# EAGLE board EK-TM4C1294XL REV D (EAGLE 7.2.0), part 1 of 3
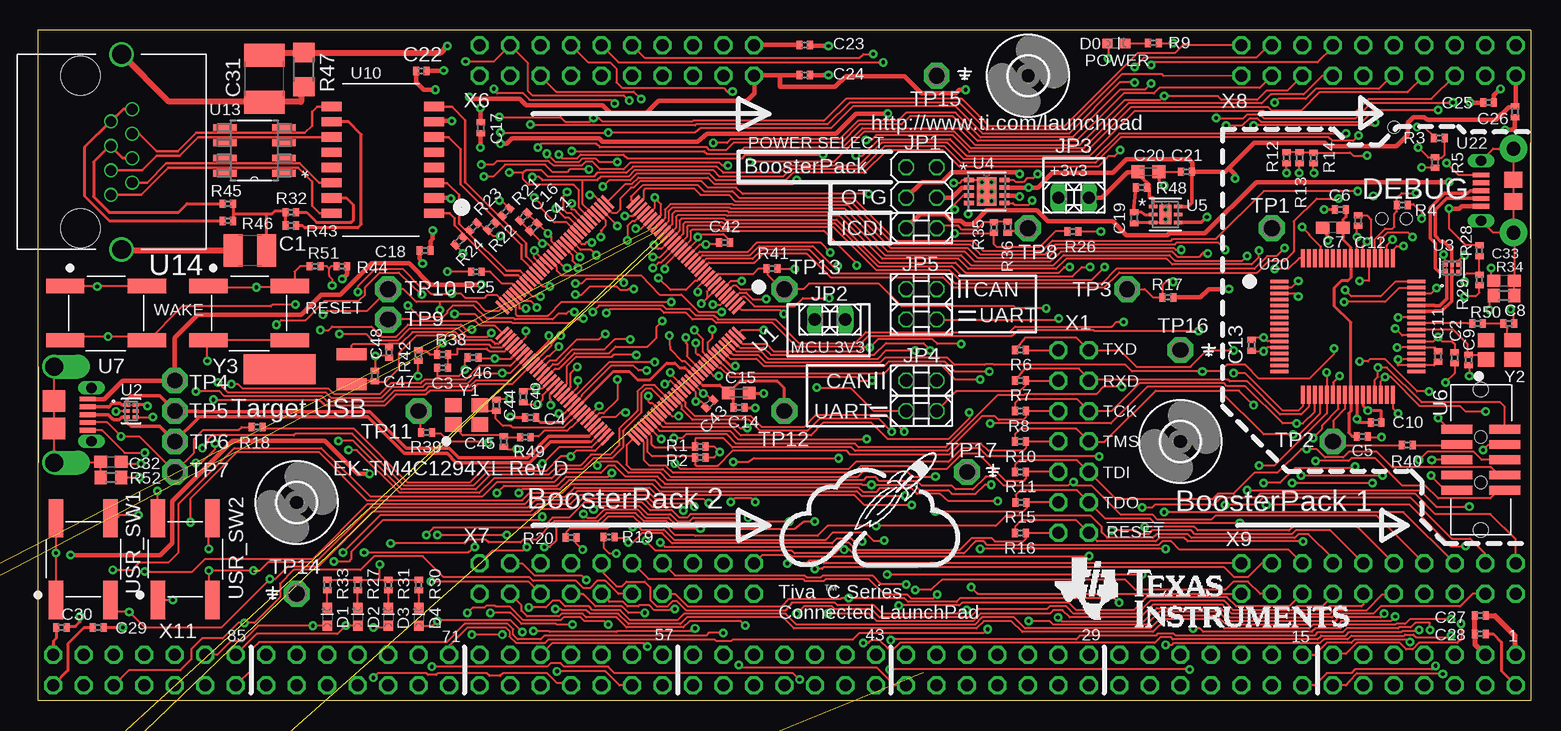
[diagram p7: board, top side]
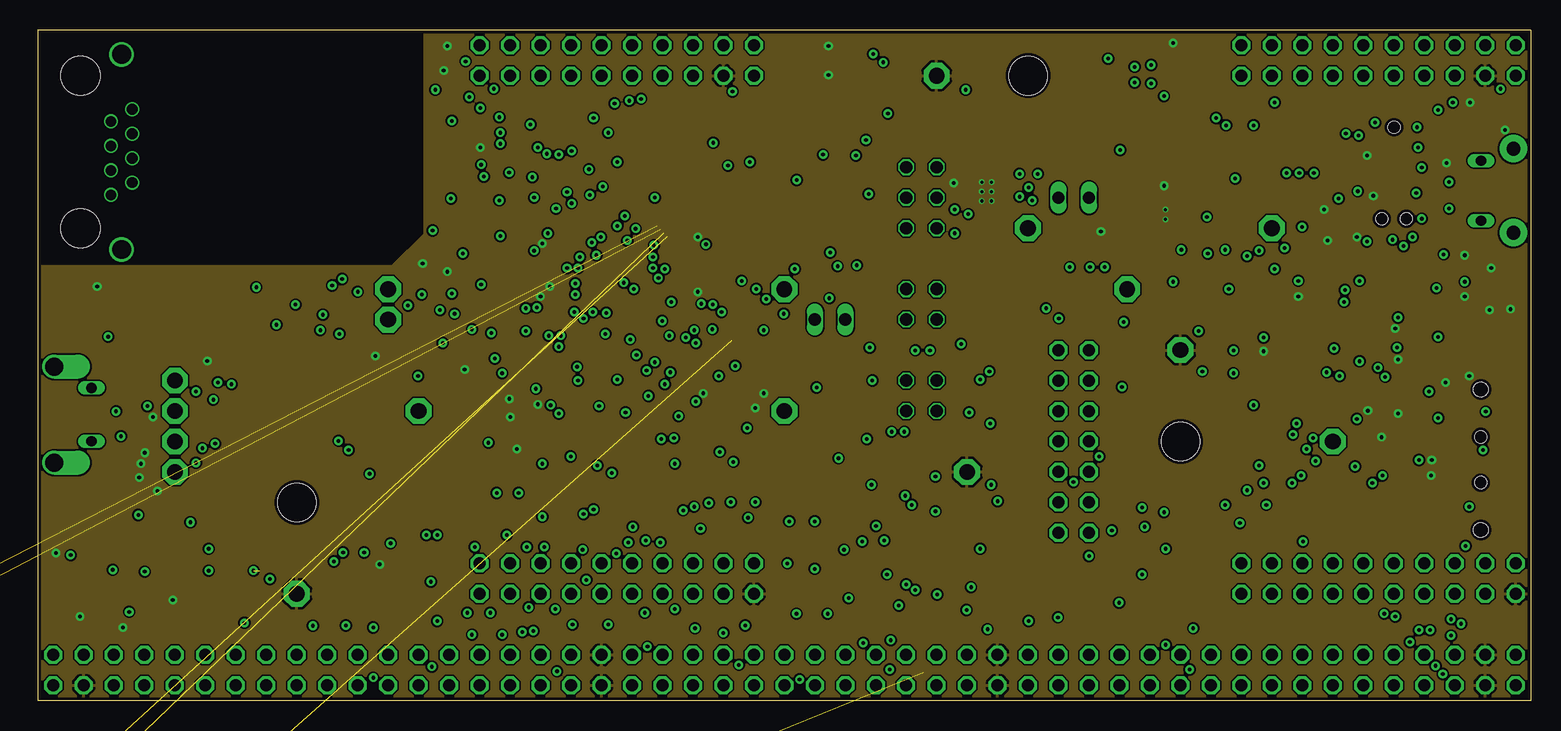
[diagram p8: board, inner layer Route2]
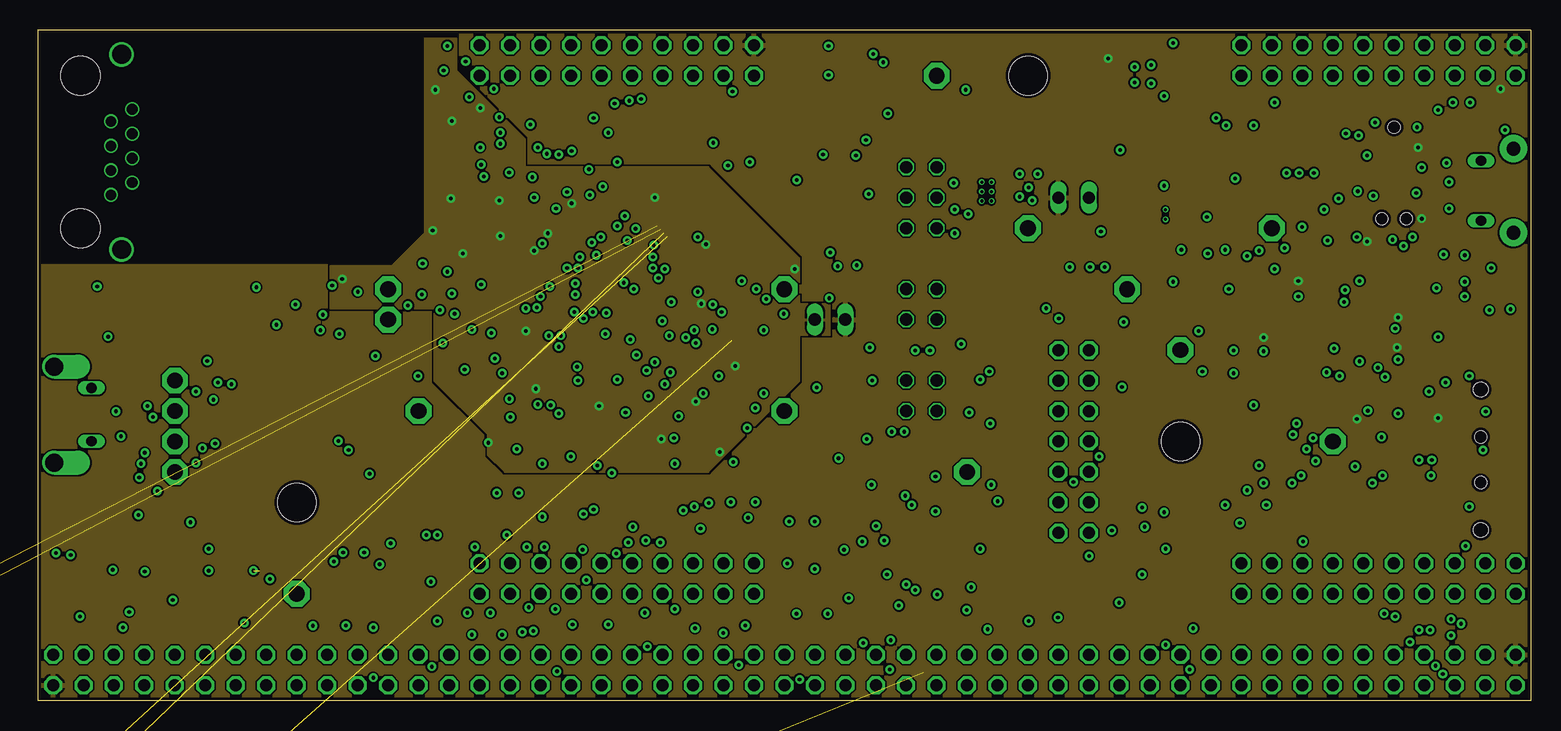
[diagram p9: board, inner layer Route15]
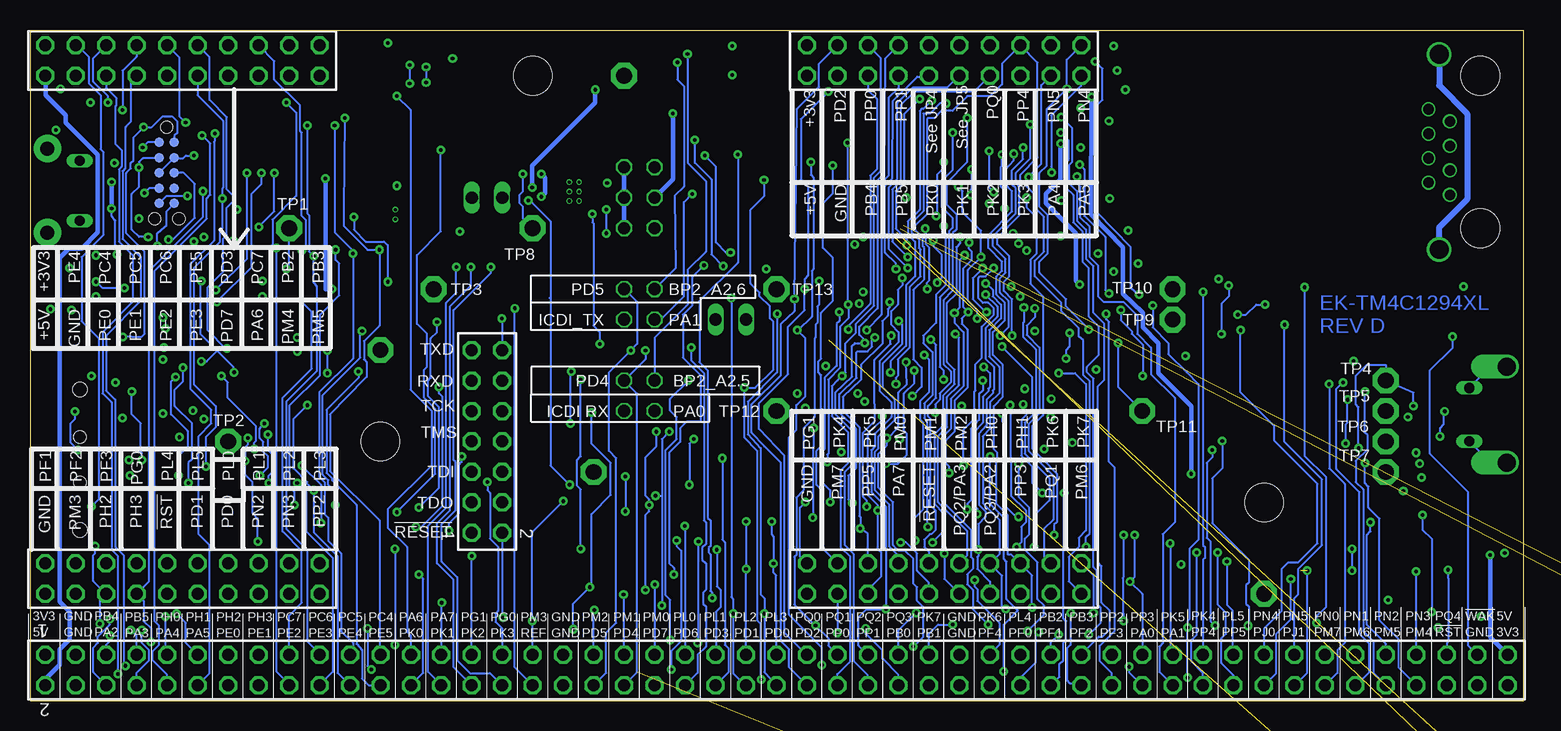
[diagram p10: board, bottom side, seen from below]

Size 124.46 x 55.88 mm. Coordinates in mm from the lower left corner, seen from the top.
Outline: 124.46,55.88 124.46,0 0,0 0,55.88 124.46,55.88
Copper layers (1+2*15+16): Top 0.035mm / dielectric 0.22mm / Route2 0.035mm / dielectric 1mm / Route15 0.035mm / dielectric 0.22mm / Bottom 0.035mm
Design rules "default *": minimum track width 6mil, minimum drill 12mil, track to track 6mil, track to pad 6mil, pad to pad 5mil, via to via 6mil, smd to smd 5mil, copper to edge 10mil, drill to drill 8mil, minimum pad ring 4mil, minimum via ring 8mil, stop-mask expansion 2mil, vias tented up to drill 13mil, thermal gap 8mil
Net classes: 1 USB: width 0.275 mm, clearance 0.152 mm; 2 Ethernet: width 0.22 mm, clearance 0.152 mm

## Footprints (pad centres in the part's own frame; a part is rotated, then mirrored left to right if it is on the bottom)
C1210 = smd 1.6 x 2.7: 1 -1.4,0; 2 1.4,0
C0402 = smd 0.5 x 0.7: 1 -0.45,0; 2 0.45,0
C0603 = smd 1.1 x 1: 1 -0.85,0; 2 0.85,0
C0603K = smd 1.05 x 1.08: 1 -0.875,0; 2 0.875,0
C1812 = smd 1.9 x 3.4: 1 -1.95,0; 2 1.95,0
CHIPLED_0603 = smd 0.8 x 0.8: A 0,-0.75; C 0,0.75
3,2 = hole 3.2: 0,0
2X03 = drill 1.016 octagon: 1 -2.54,-1.27; 2 -2.54,1.27; 3 0,-1.27; 4 0,1.27; 5 2.54,-1.27; 6 2.54,1.27
1X02 = drill 1.016 long: 1 -1.27,0; 2 1.27,0
2X02 = drill 1.016 octagon: 1 -1.27,-1.27; 2 -1.27,1.27; 3 1.27,-1.27; 4 1.27,1.27
R0402 = smd 0.5 x 0.7: 1 -0.45,0; 2 0.45,0
R0603 = smd 1 x 1.1: 1 -0.85,0; 2 0.85,0
R1206 = smd 1.6 x 1.803: 1 -1.422,0; 2 1.422,0
SWITCH_6MM_6MM_TE_CON_SMD = smd 1.2 x 3.2: P$1 4.521,6.807; P$2 4.521,0; P$3 0,6.807; P$4 0,0
P1-13 = drill 1.321 pad 2.159 octagon: TP 0,0
TQFP-128 = smd 1.45 x 0.25: P$1 0,0; P$2 0,-0.4; P$3 0,-0.8; P$4 0,-1.2; P$5 0,-1.6; P$6 0,-2; P$7 0,-2.4; P$8 0,-2.8; P$9 0,-3.2; P$10 0,-3.6; P$11 0,-4; P$12 0,-4.4; P$13 0,-4.8; P$14 0,-5.2; P$15 0,-5.6; P$16 0,-6; P$17 0,-6.4; P$18 0,-6.8; P$19 0,-7.2; P$20 0,-7.6; P$21 0,-8; P$22 0,-8.4; P$23 0,-8.8; P$24 0,-9.2; P$25 0,-9.6; P$26 0,-10; P$27 0,-10.4; P$28 0,-10.8; P$29 0,-11.2; P$30 0,-11.6; P$31 0,-12; P$32 0,-12.4; P$65 15.45,-12.4; P$66 15.45,-12; P$67 15.45,-11.6; P$68 15.45,-11.2; P$69 15.45,-10.8; P$70 15.45,-10.4; P$71 15.45,-10; P$72 15.45,-9.6; P$73 15.45,-9.2; P$74 15.45,-8.8; P$75 15.45,-8.4; P$76 15.45,-8; P$77 15.45,-7.6; P$78 15.45,-7.2; P$79 15.45,-6.8; P$80 15.45,-6.4; P$81 15.45,-6; P$82 15.45,-5.6; P$83 15.45,-5.2; P$84 15.45,-4.8; P$85 15.45,-4.4; P$86 15.45,-4; P$87 15.45,-3.6; P$88 15.45,-3.2; P$89 15.45,-2.8; P$90 15.45,-2.4; P$91 15.45,-2; P$92 15.45,-1.6; P$93 15.45,-1.2; P$94 15.45,-0.8; P$95 15.45,-0.4; P$96 15.45,0 | smd 0.25 x 1.45: P$33 1.525,-13.925; P$34 1.925,-13.925; P$35 2.325,-13.925; P$36 2.725,-13.925; P$37 3.125,-13.925; P$38 3.525,-13.925; P$39 3.925,-13.925; P$40 4.325,-13.925; P$41 4.725,-13.925; P$42 5.125,-13.925; P$43 5.525,-13.925; P$44 5.925,-13.925; P$45 6.325,-13.925; P$46 6.725,-13.925; P$47 7.125,-13.925; P$48 7.525,-13.925; P$49 7.925,-13.925; P$50 8.325,-13.925; P$51 8.725,-13.925; P$52 9.125,-13.925; P$53 9.525,-13.925; P$54 9.925,-13.925; P$55 10.325,-13.925; P$56 10.725,-13.925; P$57 11.125,-13.925; P$58 11.525,-13.925; P$59 11.925,-13.925; P$60 12.325,-13.925; P$61 12.725,-13.925; P$62 13.125,-13.925; P$63 13.525,-13.925; P$64 13.925,-13.925; P$97 13.925,1.525; P$98 13.525,1.525; P$99 13.125,1.525; P$100 12.725,1.525; P$101 12.325,1.525; P$102 11.925,1.525; P$103 11.525,1.525; P$104 11.125,1.525; P$105 10.725,1.525; P$106 10.325,1.525; P$107 9.925,1.525; P$108 9.525,1.525; P$109 9.125,1.525; P$110 8.725,1.525; P$111 8.325,1.525; P$112 7.925,1.525; P$113 7.525,1.525; P$114 7.125,1.525; P$115 6.725,1.525; P$116 6.325,1.525; P$117 5.925,1.525; P$118 5.525,1.525; P$119 5.125,1.525; P$120 4.725,1.525; P$121 4.325,1.525; P$122 3.925,1.525; P$123 3.525,1.525; P$124 3.125,1.525; P$125 2.725,1.525; P$126 2.325,1.525; P$127 1.925,1.525; P$128 1.525,1.525
DRY6 = smd 0.559 x 0.305: 1 -0.356,0.508 | smd 0.508 x 0.305: 2 -0.381,0; 3 -0.381,-0.508; 4 0.381,-0.508; 5 0.381,0; 6 0.381,0.508
DRB8_2P4X1P65 = smd 0.838 x 0.356: 1 -1.473,0.965; 2 -1.473,0.33; 3 -1.473,-0.33; 4 -1.473,-0.965; 5 1.473,-0.965; 6 1.473,-0.33; 7 1.473,0.33; 8 1.473,0.965 | smd 1.651 x 2.388: 9 0,0 | drill 0.254: V 0.406,0.787; V_2 -0.406,0; V_3 -0.406,-0.787; V_4 -0.406,0.787; V_5 0.406,-0.787; V_6 0.406,0
DRV6_1P6X1 = smd 0.711 x 0.305: 1 -1.041,0.66; 2 -1.041,0; 3 -1.041,-0.66; 4 1.041,-0.66; 5 1.041,0; 6 1.041,0.66 | smd 1.016 x 1.6: 7 0,0 | drill 0.254: V 0,-0.406; V_2 0,0.406
CON_2X5_50MIL = smd 0.74 x 2.6: P1 0,0; P2 0,4.008; P3 1.27,0; P4 1.27,4.008; P5 2.54,0; P6 2.54,4.008; P7 3.81,0; P8 3.81,4.008; P9 5.08,0; P10 5.08,4.008 | hole 1: 4.44,2; 0.64,2 | hole 1.2: 8.407,2; -3.327,2
CON_USB_MICRO_AB_HIROSE_ZX62D-AB-5P8 = smd 1.35 x 0.4: P1 2.8,1.3; P2 2.8,0.65; P3 2.8,0; P4 2.8,-0.65; P5 2.8,-1.3 | smd 1.9 x 1.8: P$1 0,-1.15; P$2 0,1.15 | drill 0.85 pad 1.092 long: P$3 3.125,2.225; P$4 3.125,-2.225 | drill 1.5 pad 2 offset: P$5 0,-4; P$6 0,4
DIL28-3 = drill 0.813 long: 1 -16.51,-3.81; 2 -13.97,-3.81; 3 -11.43,-3.81; 4 -8.89,-3.81; 5 -6.35,-3.81; 6 -3.81,-3.81; 7 -1.27,-3.81; 8 1.27,-3.81; 9 3.81,-3.81; 10 6.35,-3.81; 11 8.89,-3.81; 12 11.43,-3.81; 13 13.97,-3.81; 14 16.51,-3.81; 15 16.51,3.81; 16 13.97,3.81; 17 11.43,3.81; 18 8.89,3.81; 19 6.35,3.81; 20 3.81,3.81; 21 1.27,3.81; 22 -1.27,3.81; 23 -3.81,3.81; 24 -6.35,3.81; 25 -8.89,3.81; 26 -11.43,3.81; 27 -13.97,3.81; 28 -16.51,3.81
MAG_PULSE_HX1188FNL = smd 0.76 x 1.67: P$1 0,0; P$2 1.27,0; P$3 2.54,0; P$4 3.81,0; P$5 5.08,0; P$6 6.35,0; P$7 7.62,0; P$8 8.89,0; P$9 8.89,8.55; P$10 7.62,8.55; P$11 6.35,8.55; P$12 5.08,8.55; P$13 3.81,8.55; P$14 2.54,8.55; P$15 1.27,8.55; P$16 0,8.55
BLUETOOTH_SMD = smd 2 x 1: 1 0,0; 2 0,-1.5; 3 0,-3; 4 0,-4.5; 5 0,-6; 6 0,-7.5; 7 0,-9; 8 0,-10.5; 9 0,-12; 10 0,-13.5; 11 0,-15; 12 0,-16.5; 13 0,-18; 22 13,-18; 23 13,-16.5; 24 13,-15; 25 13,-13.5; 26 13,-12; 27 13,-10.5; 28 13,-9; 29 13,-7.5; 30 13,-6; 31 13,-4.5; 32 13,-3; 33 13,-1.5; 34 13,0 | smd 1 x 1.8: 14 1.25,-19.75; 15 2.75,-19.75; 16 4.25,-19.75; 17 5.75,-19.75; 18 7.25,-19.75; 19 8.75,-19.75; 20 10.25,-19.75; 21 11.75,-19.75
D8 = smd 1.981 x 0.559: 1 -2.464,1.905; 2 -2.464,0.635; 3 -2.464,-0.635; 4 -2.464,-1.905; 5 2.464,-1.905; 6 2.464,-0.635; 7 2.464,0.635; 8 2.464,1.905
RJ45_TE_CON_NOMAG_NOLED = drill 0.89: 1 9.93,2.54; 2 8.91,4.32; 3 7.89,2.54; 4 6.87,4.32; 5 5.85,2.54; 6 4.83,4.32; 7 3.81,2.54; 8 2.79,4.32 | drill 1.57: 9 -1.78,3.43; 10 14.48,3.43 | hole 3.25: 0,0; 12.7,0
LQFP-64-PM = smd 1.5 x 0.3: P$1 0,0; P$2 0,-0.5; P$3 0,-1; P$4 0,-1.5; P$5 0,-2; P$6 0,-2.5; P$7 0,-3; P$8 0,-3.5; P$9 0,-4; P$10 0,-4.5; P$11 0,-5; P$12 0,-5.5; P$13 0,-6; P$14 0,-6.5; P$15 0,-7; P$16 0,-7.5; P$33 11.4,-7.5; P$34 11.4,-7; P$35 11.4,-6.5; P$36 11.4,-6; P$37 11.4,-5.5; P$38 11.4,-5; P$39 11.4,-4.5; P$40 11.4,-4; P$41 11.4,-3.5; P$42 11.4,-3; P$43 11.4,-2.5; P$44 11.4,-2; P$45 11.4,-1.5; P$46 11.4,-1; P$47 11.4,-0.5; P$48 11.4,0 | smd 0.3 x 1.5: P$17 1.95,-9.45; P$18 2.45,-9.45; P$19 2.95,-9.45; P$20 3.45,-9.45; P$21 3.95,-9.45; P$22 4.45,-9.45; P$23 4.95,-9.45; P$24 5.45,-9.45; P$25 5.95,-9.45; P$26 6.45,-9.45; P$27 6.95,-9.45; P$28 7.45,-9.45; P$29 7.95,-9.45; P$30 8.45,-9.45; P$31 8.95,-9.45; P$32 9.45,-9.45; P$49 9.45,1.95; P$50 8.95,1.95; P$51 8.45,1.95; P$52 7.95,1.95; P$53 7.45,1.95; P$54 6.95,1.95; P$55 6.45,1.95; P$56 5.95,1.95; P$57 5.45,1.95; P$58 4.95,1.95; P$59 4.45,1.95; P$60 3.95,1.95; P$61 3.45,1.95; P$62 2.95,1.95; P$63 2.45,1.95; P$64 1.95,1.95
TC2030-MCP-NL = smd 0.787 x 0.787: 1 1.27,-0.635; 2 2.54,-0.635; 3 3.81,-0.635; 4 5.08,-0.635; 5 6.35,-0.635; 6 6.35,0.635; 7 5.08,0.635; 8 3.81,0.635; 9 2.54,0.635; 10 1.27,0.635 | hole 1: 0,0; 7.62,-1.016; 7.62,1.016
CON_USB_MICRO_B_FCI_10118194 = smd 1.35 x 0.4: P1 2.7,1.3; P2 2.7,0.65; P3 2.7,0; P4 2.7,-0.65; P5 2.7,-1.3 | smd 1.5 x 1.35: P6 0,0.9; P7 0,-0.9 | drill 0.85 long: P8 2.7,2.5; P9 2.7,-2.5 | drill 1.15 pad 2.286: P10 0,-3.5; P11 0,3.5
TSW-107-02-S-D = drill 1 pad 1.5 octagon: 1 7.62,-1.27; 2 7.62,1.27; 3 5.08,-1.27; 4 5.08,1.27; 5 2.54,-1.27; 6 2.54,1.27; 7 0,-1.27; 8 0,1.27; 9 -2.54,-1.27; 10 -2.54,1.27; 11 -5.08,-1.27; 12 -5.08,1.27; 13 -7.62,-1.27; 14 -7.62,1.27
TSW-110-02-S-D = drill 1 pad 1.5 octagon: 1 11.43,-1.27; 2 11.43,1.27; 3 8.89,-1.27; 4 8.89,1.27; 5 6.35,-1.27; 6 6.35,1.27; 7 3.81,-1.27; 8 3.81,1.27; 9 1.27,-1.27; 10 1.27,1.27; 11 -1.27,-1.27; 12 -1.27,1.27; 13 -3.81,-1.27; 14 -3.81,1.27; 15 -6.35,-1.27; 16 -6.35,1.27; 17 -8.89,-1.27; 18 -8.89,1.27; 19 -11.43,-1.27; 20 -11.43,1.27
TSW-149-02-S-D = drill 1 pad 1.5 octagon: 1 60.96,-1.27; 2 60.96,1.27; 3 58.42,-1.27; 4 58.42,1.27; 5 55.88,-1.27; 6 55.88,1.27; 7 53.34,-1.27; 8 53.34,1.27; 9 50.8,-1.27; 10 50.8,1.27; 11 48.26,-1.27; 12 48.26,1.27; 13 45.72,-1.27; 14 45.72,1.27; 15 43.18,-1.27; 16 43.18,1.27; 17 40.64,-1.27; 18 40.64,1.27; 19 38.1,-1.27; 20 38.1,1.27; 21 35.56,-1.27; 22 35.56,1.27; 23 33.02,-1.27; 24 33.02,1.27; 25 30.48,-1.27; 26 30.48,1.27; 27 27.94,-1.27; 28 27.94,1.27; 29 25.4,-1.27; 30 25.4,1.27; 31 22.86,-1.27; 32 22.86,1.27; 33 20.32,-1.27; 34 20.32,1.27; 35 17.78,-1.27; 36 17.78,1.27; 37 15.24,-1.27; 38 15.24,1.27; 39 12.7,-1.27; 40 12.7,1.27; 41 10.16,-1.27; 42 10.16,1.27; 43 7.62,-1.27; 44 7.62,1.27; 45 5.08,-1.27; 46 5.08,1.27; 47 2.54,-1.27; 48 2.54,1.27; 49 0,-1.27; 50 0,1.27; 51 -2.54,-1.27; 52 -2.54,1.27; 53 -5.08,-1.27; 54 -5.08,1.27; 55 -7.62,-1.27; 56 -7.62,1.27; 57 -10.16,-1.27; 58 -10.16,1.27; 59 -12.7,-1.27; 60 -12.7,1.27; 61 -15.24,-1.27; 62 -15.24,1.27; 63 -17.78,-1.27; 64 -17.78,1.27; 65 -20.32,-1.27; 66 -20.32,1.27; 67 -22.86,-1.27; 68 -22.86,1.27; 69 -25.4,-1.27; 70 -25.4,1.27; 71 -27.94,-1.27; 72 -27.94,1.27; 73 -30.48,-1.27; 74 -30.48,1.27; 75 -33.02,-1.27; 76 -33.02,1.27; 77 -35.56,-1.27; 78 -35.56,1.27; 79 -38.1,-1.27; 80 -38.1,1.27; 81 -40.64,-1.27; 82 -40.64,1.27; 83 -43.18,-1.27; 84 -43.18,1.27; 85 -45.72,-1.27; 86 -45.72,1.27; 87 -48.26,-1.27; 88 -48.26,1.27; 89 -50.8,-1.27; 90 -50.8,1.27; 91 -53.34,-1.27; 92 -53.34,1.27; 93 -55.88,-1.27; 94 -55.88,1.27; 95 -58.42,-1.27; 96 -58.42,1.27; 97 -60.96,-1.27; 98 -60.96,1.27
NDK3.2X2.5 = smd 1.4 x 1.2: P$1 0,0; P$2 2.2,0; P$3 2.2,1.6; P$4 0,1.6
CRYSTAL_32K_SMD = smd 2.5 x 1: P$1 0,1.25; P$2 0,-1.25 | smd 6 x 2.5: P$3 -6,0

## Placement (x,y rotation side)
C1  1000pF  [C1210]  17.68,37.49 180 top
C2  0.1uF  [C0402]  118.11,28.57 270 top
C3  0.1uF  [C0402]  33.76,27.74 180 top
C4  0.1uF  [C0402]  41.07,23.6 180 top
C5  0.1uF  [C0402]  110.41,22 0 top
C6  1.0uF  [C0402]  108.58,40.92 180 top
C7  2.2uF  [C0603]  107.95,39.42 180 top
C8  12pF  [C0402]  122.63,31.42 0 top
C9  12pF  [C0402]  119.25,28.37 270 top
C10  0.1uF  [C0402]  111.56,23.16 0 top
C11  0.1uF  [C0402]  116.71,28.68 270 top
C12  0.1uF  [C0402]  110.06,40.01 270 top
C13  0.1uF  [C0402]  101.17,29.62 270 top
C14  1.0uF  [C0402]  58.45,24.41 0 top
C15  2.2uF  [C0603K]  58.45,25.63 0 top
C16  0.1uF  [C0402]  40.49,40.31 225 top
C17  0.1uF  [C0402]  36.93,47.73 270 top
C18  0.1uF  [C0402]  32.28,37.49 180 top
C19  0.1uF  [C0402]  91.39,40.23 270 top
C20  2.2uF  [C0603K]  92.58,44.07 0 top
C21  0.1uF  [C0402]  95.76,44.07 180 top
C22  0.1uF  [C0402]  31.98,52.48 0 top
C23  0.1uF  [C0402]  63.93,54.64 0 top
C24  0.1uF  [C0402]  63.93,52.12 0 top
C25  0.1uF  [C0402]  120.93,49.83 180 top
C26  0.1uF  [C0402]  123.14,49.07 270 top
C27  0.1uF  [C0402]  120.24,7.09 180 top
C28  0.1uF  [C0402]  120.24,5.56 180 top
C29  0.1uF  [C0402]  5.03,6.1 0 top
C30  0.1uF  [C0402]  1.98,6.1 0 top
C31  4700pF  [C1812]  18.9,51.82 90 top
C32  3300pF  [C0603]  6.1,19.89 0 top
C33  3300pF  [C0603]  122.22,34.98 180 top
C40  0.1uF  [C0402]  40.46,25.32 270 top
C41  0.1uF  [C0402]  41.33,39.45 225 top
C42  0.1uF  [C0402]  57.25,38.18 0 top
C43  0.1uF  [C0402]  56.01,24.74 45 top
C44  12pF  [C0402]  38.23,24.61 90 top
C45  12pF  [C0402]  38.84,21.59 270 top
C46  0.1uF  [C0402]  36.3,28.6 180 top
C47  12pF  [C0402]  28.09,27.05 90 top
C48  12pF  [C0402]  29.29,29.01 270 top
D0  [CHIPLED_0603]  89.92,54.76 270 top
D1  [CHIPLED_0603]  24.13,6.99 0 top
D2  [CHIPLED_0603]  26.67,6.99 0 top
D3  [CHIPLED_0603]  29.21,6.99 0 top
D4  [CHIPLED_0603]  31.75,6.99 0 top
H1  MOUNT-HOLE3.2  [3,2]  95.25,21.59 0 top
H4  MOUNT-HOLE3.2  [3,2]  21.59,16.51 0 top
H6  MOUNT-HOLE3.2  [3,2]  82.55,52.07 0 top
J1  [JUMP]  73.66,39.37 90 top
J2  [JUMP]  73.66,24.13 90 top
J3  [JUMP]  86.36,41.91 90 top
J4  [JUMP]  73.66,26.67 90 top
J5  [JUMP]  73.66,31.75 90 top
J6  [JUMP]  73.66,34.29 90 top
J7  [JUMP]  66.04,31.75 90 top
JP1  [2X03]  73.66,41.91 270 top
JP2  [1X02]  66.04,31.75 180 top
JP3  [1X02]  86.36,41.91 0 top
JP4  [2X02]  73.66,25.4 90 top
JP5  [2X02]  73.66,33.02 90 top
R1  10k  [R0402]  55.22,21.18 180 top
R2  10k  [R0402]  55.22,20.24 180 top
R3  10k  [R0402]  116.84,46.89 0 top
R4  10k  [R0402]  113.74,41.3 180 top
R5  10k  [R0402]  116.48,44.83 270 top
R6  0  [R0402]  81.92,29.21 180 top
R7  0  [R0402]  81.92,26.67 180 top
R8  0  [R0402]  81.92,24.13 180 top
R9  330  [R0402]  92.99,54.81 180 top
R10  0  [R0402]  81.92,21.59 180 top
R11  0  [R0402]  81.92,19.05 180 top
R12  5.6k  [R0402]  104.09,45.24 90 top
R13  5.6k  [R0402]  105.18,45.24 90 top
R14  5.6k  [R0402]  106.35,45.21 90 top
R15  0  [R0402]  81.97,16.51 180 top
R16  0  [R0402]  81.92,13.97 180 top
R17  100k  [R0402]  94.21,33.6 180 top
R18  100  [R0402]  18.29,22.78 180 top
R19  0  [R0402]  47.62,13.61 0 top
R20  0  [R0402]  44.45,13.59 180 top
R21  49.9  [R0402]  39.01,40.72 225 top
R22  49.9  [R0402]  37.82,39.52 45 top
R23  49.4  [R0402]  36.3,39.47 225 top
R24  49.9  [R0402]  35.1,38.28 45 top
R25  4.87k 1%  [R0402]  36.55,35.74 180 top
R26  100k  [R0402]  86.28,39.09 0 top
R27  330  [R0402]  26.67,9.63 270 top
R28  5.6k  [R0402]  120.17,37.49 90 top
R29  10k  [R0402]  120.17,35.05 90 top
R30  330  [R0402]  31.75,9.63 270 top
R31  330  [R0402]  29.21,9.63 270 top
R32  75  [R0402]  21.11,40.69 0 top
R33  330  [R0402]  24.13,9.63 270 top
R34  1M  [R0603]  122.22,33.76 0 top
R35  10k  [R0402]  79.71,39.42 270 top
R36  100k  [R0402]  80.85,39.45 90 top
R38  51  [R0402]  33.76,28.83 0 top
R39  0  [R0402]  32.41,22.33 0 top
R40  0  [R0402]  114.17,21.29 0 top
R41  0  [R0402]  61.21,36.02 0 top
R42  1M  [R0402]  31.72,28.75 270 top
R43  75  [R0402]  21.11,39.57 0 top
R44  10k  [R0402]  25.35,36.2 180 top
R45  75  [R0402]  15.85,41.4 180 top
R46  75  [R0402]  15.85,39.98 180 top
R47  1M  [R1206]  22.17,52.58 270 top
R48  [R0402]  92,42.76 0 top
R49  2k  [R0402]  40.64,21.95 0 top
R50  2k  [R0402]  120.02,31.42 0 top
R51  100  [R0402]  23.13,36.2 0 top
R52  1M  [R0603]  6.1,18.59 180 top
RESET  SWITCH_TACTILE  [SWITCH_6MM_6MM_TE_CON_SMD]  14.22,34.54 270 top
TP1  TPPAD1-13  [P1-13]  102.87,39.37 270 top
TP2  TPPAD1-13  [P1-13]  107.95,21.59 0 top
TP3  TPPAD1-13  [P1-13]  90.81,34.29 180 top
TP4  TPPAD1-13  [P1-13]  11.43,26.67 90 top
TP5  TPPAD1-13  [P1-13]  11.43,24.13 270 top
TP6  TPPAD1-13  [P1-13]  11.43,21.59 90 top
TP7  TPPAD1-13  [P1-13]  11.43,19.05 270 top
TP8  TPPAD1-13  [P1-13]  82.55,39.37 180 top
TP9  TPPAD1-13  [P1-13]  29.21,31.75 0 top
TP10  TPPAD1-13  [P1-13]  29.21,34.29 0 top
TP11  TPPAD1-13  [P1-13]  31.75,24.13 0 top
TP12  TPPAD1-13  [P1-13]  62.23,24.13 0 top
TP13  TPPAD1-13  [P1-13]  62.23,34.29 0 top
TP14  TPPAD1-13  [P1-13]  21.59,8.89 0 top
TP15  TPPAD1-13  [P1-13]  74.93,52.07 0 top
TP16  TPPAD1-13  [P1-13]  95.25,29.21 0 top
TP17  TPPAD1-13  [P1-13]  77.47,19.05 0 top
U1  TM4C1294NCPDT  [TQFP-128]  58.42,32.77 225 top
U2  TPD4S012_DRY_6  [DRY6]  7.77,24.13 0 top
U3  TPD4S012_DRY_6  [DRY6]  117.88,36.04 90 top
U4  TPS2052B_DRB_8  [DRB8_2P4X1P65]  79.1,42.42 0 top
U5  TPS73733_DRV_6  [DRV6_1P6X1]  94,40.5 0 top
U6  JTAG_ARM_10PIN  [CON_2X5_50MIL]  118.29,22.61 270 top
U7  CON_USB_HIROSE_MICRO_AB_ZX62D_AB_5P8  [CON_USB_MICRO_AB_HIROSE_ZX62D-AB-5P8]  1.35,23.83 0 top
U8  ATMEGA328P_PDIP  [DIL28-3]  not placed on the board
U9  ATMEGA328P_PDIP  [DIL28-3]  not placed on the board
U10  MAG_PULSE_HX1188FNL  [MAG_PULSE_HX1188FNL]  33.05,40.61 90 top
U11  HC_05  [BLUETOOTH_SMD]  not placed on the board
U13  SLVU2.8-4  [D8]  18.06,45.85 180 top
U14  JACK_RJ45_NOMAG_NOLED_TECON  [RJ45_TE_CON_NOMAG_NOLED]  3.56,52.07 270 top
U20  TM4C123GH6PMI  [LQFP-64-PM]  103.5,34.92 0 top
U21  TC2050-NL-MCP-NL  [TC2030-MCP-NL]  113.06,47.78 270 bottom
U22  CON_USB_FCI_MICRO_B_10118194  [CON_USB_MICRO_B_FCI_10118194]  123.01,42.49 180 top
USR_SW1  SWITCH_TACTILE  [SWITCH_6MM_6MM_TE_CON_SMD]  1.52,8.38 0 top
USR_SW2  SWITCH_TACTILE  [SWITCH_6MM_6MM_TE_CON_SMD]  10.03,8.38 0 top
WAKE  SWITCH_TACTILE  [SWITCH_6MM_6MM_TE_CON_SMD]  2.29,34.54 270 top
X1  TSW-107-02-S-D  [TSW-107-02-S-D]  86.36,21.59 270 bottom
X6  TSW-110-02-S-D  [TSW-110-02-S-D]  48.26,53.34 180 bottom
X7  TSW-110-02-S-D  [TSW-110-02-S-D]  48.26,10.16 180 bottom
X8  TSW-110-02-S-D  [TSW-110-02-S-D]  111.76,53.34 180 bottom
X9  TSW-110-02-S-D  [TSW-110-02-S-D]  111.76,10.16 180 bottom
X11  TSW-149-02-S-D  [TSW-149-02-S-D]  62.23,2.54 180 bottom
Y1  25Mhz  [NDK3.2X2.5]  34.65,23.01 0 top
Y2  16M  [NDK3.2X2.5]  120.73,28.42 0 top
Y3  CRYATL_32K_SMD  [CRYSTAL_32K_SMD]  26.16,27.61 0 top

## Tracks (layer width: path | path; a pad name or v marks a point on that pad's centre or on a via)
!DEBUG_RESET_OUT  (via drill 0.3)
  Top 0.152: U20.P$23 108.43,25.45 108.43,24.31 107.06,22.94 107.06,22.63 v106.3,21.87 | R16.2 81.46,13.95 81.46,14.48 81.49,14.51 81.99,15.01 86.59,15.01 X1.1 87.61,13.97 88.32,13.26 93.19,13.26 93.5,13.56 95.56,13.56 95.86,13.26 v105.46,13.26 | U6.P10 121.77,17.53 121.08,16.84 116.74,16.84 115.67,17.91 113.77,17.91 111.48,20.19 109.5,20.19 109.27,19.96 v106.53,19.96
  Bottom 0.152: v105.46,13.26 105.46,15.16 105.92,15.62 105.92,18.21 106.53,18.82 v106.53,19.96 106.53,21.11 106.3,21.34 v106.3,21.87
!EXTERNAL_DEBUG
  Top 0.152: U20.P$24 108.95,24.3 107.97,23.32 107.97,21.61 | 107.97,21.61 TP2.TP | 107.97,21.61 108.33,21.26 113.5,21.26 R40.1
!HIB
  Top 0.152: TP9.TP 29.34,31.77 31.01,31.77 31.17,31.62 36.5,31.62 36.88,31.24 38.1,31.24 38.12,31.22 U1.P$65
!TARGET_RESET  (via drill 0.3)
  Top 0.152: RESET.P$4 15.54,34.52 15.24,34.52 15.32,34.44 v18.21,34.44 | v18.21,34.44 18.25,34.48 19.62,34.48 20.01,34.78 | 20.01,34.78 RESET.P$3 | v51.89,13.18 52.27,12.8 66.45,12.8 66.83,13.18 67.59,13.18 68.2,12.57 76.89,12.57 77.88,13.56 79.48,13.56 79.78,13.26 82.14,13.26 82.37,13.49 82.37,13.79 R16.1 X1.2 | v85.04,6.93 85.34,6.63 92.2,6.63 93.27,7.7 98.6,7.7 99.36,6.93 105.31,6.93 105.61,7.24 107.75,7.24 108.05,7.54 110.8,7.54 112.09,8.84 112.98,8.84 X9.10 | X7.10 48.41,8.89 47.32,9.98 46.63,9.98 46.02,9.37 45.49,9.37 44.88,9.98 41.3,9.98 41,10.29 33.83,10.29 32.08,12.04 28.04,12.04 26.9,10.9 21.34,10.9 20.19,9.75 20.19,8.61 18.06,6.48 v17.22,6.48 16.69,6.48 15.39,5.18 13.72,5.18 12.8,4.27 12.8,3.43 11.89,2.52 7.59,2.52 X11.94 | v18.22,34.44 v18.21,34.44 | R51.1 21.87,36.2 21.41,35.74 21.41,34.98 21.38,34.86 21.38,34.4 21.79,34.82 20.01,34.78
  Bottom 0.152: v51.89,13.18 51.44,13.18 50.52,12.27 50.52,10.82 49.53,9.83 X7.10 | X1.2 85.09,6.99 v85.04,6.93 | v18.21,34.44 18.21,20.42 16.46,18.67 16.46,7.77 17.22,7.01 v17.22,6.48
!TARGET_RESET_FILTERED  (via drill 0.3)
  Top 0.152: 39.55,28.6 | C46.1 36.88,28.5 v38.1,28.5 39.45,28.5 39.55,28.6 | R44.2 24.46,36.2 24.31,36.04 24.31,35.97 | v24.54,34.59 24.54,35.13 24.31,35.36 24.31,35.42 24.31,35.97 | v25.15,30.56 27.36,30.56 27.89,30.02 30.02,30.02 31.01,31.01 35.05,31.01 35.74,30.33 37.49,30.33 v37.8,30.63 | 24.31,35.97 24.08,36.2 23.77,36.2 23.79,36.19 R51.2 | U1.P$70 39.55,28.6
  Bottom 0.152: v24.54,34.59 24.54,33.68 25.15,33.07 v25.15,30.56 | v37.8,30.63 37.8,29.52 38.1,29.21 v38.1,28.5
!WAKE  (via drill 0.3)
  Top 0.152: WAKE.P$2 2.9,30.33 4.88,30.32 v5.87,30.32 8.38,30.32 8.84,29.79 WAKE.P$1 9.02,30.28 9.07,29.87 12.04,32.84 19.43,32.84 19.58,32.99 v21.49,32.99 | 33.53,33.22 36.58,33.22 37.34,32.46 38.42,32.46 U1.P$64 | 33.53,33.22 31.55,33.22 30.48,34.29 TP10.TP 29.21,34.24 27.43,32.46 24.08,32.46 v23.77,32.16 | v33.53,32.54 33.53,33.22 | v31.7,27.05 31.73,27.08 R42.2
  Bottom 0.152: X11.95 4.57,4.57 4.57,17.37 7.77,20.57 7.77,27.51 5.87,29.41 v5.87,30.32 | v23.77,32.16 23.09,32.16 22.25,32.99 v21.49,32.99 | v33.53,32.54 33.53,31.7 32.61,30.79 32.61,30.56 31.7,29.64 v31.7,27.05
+3V3  (via drill 0.3)
  Top 0.152: D0.A 89.23,54.76 v89.23,53.49 | U20.P$42 114.53,31.93 v113.39,31.93 | U20.P$54 110.45,37.91 v110.8,38.25 111.18,38.63 111.18,40.08 110.87,40.39 110.19,40.39 110.19,40.31 110.22,40.43 C12.1 | v115.06,46.1 115.9,45.26 116.51,45.26 R5.1 116.5,45.25 117.03,45.25 117.27,45.49 117.27,46.79 117.2,46.86 R3.2 | v115.37,40.16 115.37,40.69 114.68,41.38 114.3,41.38 114.27,41.38 R4.1 | U20.P$2 104.53,34.42 v105.08,34.98 | 116.48,29.18 C11.1 116.42,29.43 U20.P$37 113.31,29.43 v113.31,29.41 | U20.P$11 102.51,29.93 v102.18,30.25 102.17,30.27 101.51,30.27 101.35,30.1 C13.1 | U6.P1 117.68,22.61 v116.74,23.55
  Top 0.254: C29.1 4.38,6.06 3.85,6.06 2.52,4.72 2.52,2.52 X11.98 | U20.P$26 109.95,23.85 v109.96,23.47 109.96,23.24 110.03,23.16 C10.1
  Top 0.381: C23.1 59.72,54.63 X6.1 | C25.1 121.38,50.44 v121.92,50.98
  Top 0.406: C27.1 121.46,7.09 123.14,5.41 123.14,3.81 123.11,3.95 X11.1
  Bottom 0.152: U21.1 114.66,46.51 v115.06,46.1 | v105.08,34.98 105,34.9 | v113.31,29.41 113.39,29.41 | v116.74,23.55 116.74,23.47
  Bottom 0.381: v121.92,50.98 121.92,51.05
  pour Route15 (rank 2): 32.26,55.88 124.46,55.88 124.46,0 0,0 0,36.2 29.51,36.2 32.26,38.91
+5V  (via drill 0.3)
  Top 0.254: C30.1 1.53,5.19 1.29,4.95 1.29,3.96 1.22,3.89 1.33,3.87 X11.97 | X11.2 122,2.46 122,4.88 121.31,5.56 C28.1
  Top 0.305: U5.6 95.88,41.16 95.86,41.15 96.21,41.5 C21.1
  Top 0.356: U4.7 v82.6,42.75
  Top 0.381: 123.17,52.07 X8.2 123.19,49.77 C26.1 122.87,49.45 122.61,49.45 121.54,48.39 115.82,48.39 115.59,48.62 114.68,48.62 114.22,48.16 114.22,47.17 113.23,46.18 107.59,46.18 107.29,46.48 101.42,46.48 99.29,44.35 | 99.29,44.35 99.01,44.07 C21.1 96.24,44.12 96.24,44.81 95.94,45.11 90.75,45.11 89.61,43.97 84.58,43.97 83.36,42.75 v82.6,42.75 | R17.1 96.93,33.6 97.61,34.29 v99.29,34.29 | v99.82,43.51 99.82,43.81 99.29,44.35 | v77.34,50.9 76.81,50.9 76.53,50.62 73.66,50.62 72.24,52.05 67.36,52.05 66.45,51.13 61.87,51.13 61.87,52.12 | v2.74,12.12 10.21,12.12 11.2,13.11 11.2,16.61 16.23,21.64 23.93,21.64 26.67,18.9 v27.66,18.9 | v35.97,50.29 36.12,50.14 40.16,50.14 40.69,49.61 47.09,49.61 47.7,49 50.75,49 51.74,49.99 59.13,49.99 59.74,50.6 59.74,52.02 X6.2 59.74,52.12 61.87,52.12 | C24.1 61.87,52.12
  Bottom 0.381: v99.29,34.29 99.82,34.29 v99.82,43.51 | v77.34,50.9 77.34,49.84 82.6,44.58 v82.6,42.75 | X11.97 2.74,5.28 v2.74,12.12 | v35.97,50.29 36.04,40.54 33.38,37.8 33.38,33.91 31.7,32.31 31.7,31.09 30.4,29.79 30.4,27.28 27.66,24.54 v27.66,18.9 | X11.2 123.19,1.78 122,2.97 122,4.27 121.16,5.11 121.16,7.39 122,8.23 122,36.88 121.23,37.64 120.17,37.64 118.8,39.01 118.8,45.49 121.46,48.16 121.46,48.77 123.14,50.44 123.14,52.02 X8.2
BP2_A2.5  (via drill 0.3)
  Top 0.152: X6.9 50.57,53.57 68.5,53.57 68.81,53.87 v69.65,53.87
  Bottom 0.152: v69.65,53.87 69.65,44.81 68.12,43.28 68.12,37.41 69.65,35.89 69.65,32.99 72.39,30.25 JP4.4
BP2_A2.6  (via drill 0.3)
  Top 0.152: X6.11 48.41,53.19 v70.48,53.19
  Bottom 0.152: v70.48,53.19 70.48,51.74 69.95,51.21 69.95,42.82 70.71,42.06 70.64,36.04 JP5.4
CHASSIS
  Top 0.508: C1.2 7.09,37.49 U14.10 | U14.9 10.93,49.91 17.91,49.91 C31.1 20.06,49.89 21.95,49.89 21.95,50.83 22.1,50.83 | R47.2 21.84,51.05 22.1,50.8 22.1,50.83 | 22.1,51.05 22.1,50.83
  Bottom 0.508: U14.9 6.99,51.26 4.65,48.92 4.65,41.76 7.01,39.4 7.01,37.61 U14.10
DEBUG_ACTIVE  (via drill 0.3)
  Top 0.152: v103.1,35.97 104.24,35.97 105.15,36.88 U20.P$64
  Bottom 0.152: v103.1,35.97 102.87,36.2 TP1.TP
DEBUG_PC0/TCK/SWCLK  (via drill 0.3)
  Top 0.152: U20.P$19 106.45,24.08 105.46,23.09 v104.93,23.09 103.78,23.09 100.66,26.21 99.14,26.21 98.91,26.44 91.82,26.44 89.51,24.13 X1.9 86.61,25.15 81.84,25.15 81.49,24.8 81.49,24.19 81.38,24.08 | R8.2 81.38,24.08 | 81.38,24 81.38,24.08 | v112.09,18.75 v105.31,18.75 | U20.P$30 111.95,26.61 v112.32,26.98 112.78,26.98 115.21,24.54 118.57,24.54 119.02,24.08 v120.7,24.08 | U6.P4 121.84,21.34 121.69,21.26 120.85,21.26 v120.47,20.88
  Bottom 0.152: v105.31,18.75 104.62,19.43 104.62,20.34 105,20.73 105,21.57 105.31,21.87 105.31,22.63 v104.93,23.09 | v112.09,18.75 112.09,20.42 111.33,21.11 111.33,22.48 112.7,23.85 112.7,26.59 v112.32,26.98 | v120.47,20.88 121.08,21.49 121.08,23.09 120.7,23.47 v120.7,24.08
DEBUG_PC1/TMS/SWDIO  (via drill 0.3)
  Top 0.152: U20.P$20 106.91,25.43 106.91,23.93 105.16,22.17 v104.62,22.17 102.18,22.17 98.53,25.83 93.19,25.83 88.92,21.57 87.94,21.57 87.86,21.64 X1.7 87.61,21.59 86.56,22.63 81.92,22.63 81.46,22.17 81.46,21.79 81.53,21.72 R10.2 | v104.55,18.14 v111.25,18.14 | U20.P$29 111.45,26.72 111.71,26.98 v111.71,27.74 112.47,27.74 115.37,24.84 121.92,24.84 122.3,24.46 U6.P2
  Bottom 0.152: v104.55,18.14 104.55,18.75 104.24,19.05 104.24,20.5 104.62,20.88 v104.62,22.17 | v111.25,18.14 111.25,19.81 110.95,20.12 110.95,23.09 112.39,24.54 112.39,25.91 111.71,26.59 v111.71,27.74
DEBUG_PC2/TDI  (via drill 0.3)
  Top 0.152: X1.5 87.63,19.13 | 107.9,25.42 U20.P$22 107.97,25.5 107.97,26.52 v108.51,27.05 | X1.5 86.64,20.04 82.26,20.04 81.84,20.04 81.46,19.66 81.46,19.13 R11.2 | X1.5 89.92,16.76 97.92,16.76 98.37,17.22 99.67,17.22 101.42,18.97 103.33,18.97 105.31,20.95 v105.77,20.95 106.6,20.95 107.29,20.27 108.81,20.27 109.27,20.73 111.63,20.73 112.93,19.43 121.16,19.43 121.79,18.8 U6.P8
  Bottom 0.152: v108.51,27.05 107.97,26.52 107.97,25.22 105.61,22.86 105.61,21.64 105.77,21.49 v105.77,20.95
DEBUG_PC3/TDO/SWO  (via drill 0.3)
  Top 0.152: X1.3 87.76,16.51 | X1.3 87.63,16.54 86.64,17.53 81.92,17.53 81.53,17.14 81.53,16.61 R15.2 | 88.06,16.46 X1.3 | 87.94,16.46 87.88,16.51 X1.3 | v101.8,19.58 103.1,19.58 107.45,23.94 U20.P$21 107.44,25.49 v107.44,27.36 | v100.2,14.78 93.12,14.78 92.73,15.16 88.98,15.16 X1.3 | U20.P$53 110.95,34.98 v110.19,34.98 | v115.98,25.76 114.99,25.76 112.32,28.42 111.02,28.42 110.87,28.27 v110.19,28.27 | U6.P6 120.37,20.07 119.71,20.73 115.82,20.73 v115.14,20.04
  Bottom 0.152: v101.8,19.58 100.2,17.98 v100.2,14.78 | v110.19,34.98 110.26,34.9 110.26,30.56 108.85,29.15 | 108.85,29.15 107.52,27.81 107.52,27.43 v107.44,27.36 | v110.19,28.27 109.73,28.27 108.85,29.15 | v115.14,20.04 115.14,20.65 115.21,20.73 115.21,23.09 115.98,23.85 v115.98,25.76
DEBUG_VBUS  (via drill 0.3)
  Top 0.152: U3.6 117.35,36.42 117.35,37.11 v117.2,37.19 | R28.2 120.13,38.1 120.02,37.95 119.02,37.95 117.65,39.32 v117.65,41
  Top 0.381: JP1.5 72.39,39.4 73.53,40.54 75.67,40.54 76.2,40.01 76.96,40.01 77.27,39.7 77.95,39.7 79.1,40.84 83.29,40.84 84.2,39.93 89.61,39.93 90.75,38.79 94.18,38.79 94.34,38.94 97.31,38.94 101.58,43.2 v117.65,43.2 | U22.P1 118.69,41.19 118.49,41 v117.65,41
  Bottom 0.152: v117.2,37.19 117.2,37.8 117.35,37.95 117.35,40.01 117.65,40.39 v117.65,41
  Bottom 0.381: v117.65,41 v117.65,43.2
EN0RXI_N
  Top 0.22: 38.56,40.24 40.7,38.1 40.7,37.01 U1.P$53 | 38.56,40.24 35.62,43.18 35.62,48.38 34.52,49.48 33.07,49.48 U10.P$8 | R21.2 38.61,40.24 38.56,40.24
EN0RXI_P
  Top 0.22: 38.3,39.98 40.33,37.95 40.33,36.82 U1.P$54 | 38.3,39.98 35.25,43.03 35.25,45.93 34.24,46.94 33.07,46.94 U10.P$6 | R22.2 38.3,39.92 38.3,39.98
EN0TXO_N
  Top 0.152: 40.98,35.03 40.21,35.8
  Top 0.22: 40.21,35.8 39.07,35.8 35.79,39.07 | 35.79,39.07 35.11,39.75 35.11,42.16 34.14,43.13 33.07,43.13 U10.P$3 | R23.2 35.82,39.07 35.79,39.07 | U1.P$56 40.98,35.03
EN0TXO_P
  Top 0.152: 40.71,34.77 40.05,35.42
  Top 0.22: 40.05,35.42 38.91,35.42 35.49,38.84 | 35.49,38.84 34.74,39.6 34.74,40.19 34.34,40.59 33.07,40.59 U10.P$1 | R24.2 35.49,38.74 35.49,38.84 | U1.P$57 40.71,34.77
GND  (via drill 0.3)
  Top 0.152: C43.2 56.08,25.15 55.63,25.6 v55.47,25.6 54.46,26.62 U1.P$114 | U4.1 79.1,43.38 U4.9 U4.V_2 78.64,42.42 78.64,43.2 78.64,43.36 77.04,43.36 76.81,43.13 v76.35,43.13 | U2.4 v9.6,23.62 | C48.2 29.25,28.49 29.34,28.42 29.03,28.73 v28.14,28.73 | v28.14,28.73 28.2,28.66 | C47.2 28.14,27.62 v28.14,28.73 | R26.2 v88.62,39.09 | C20.2 C21.2 | R9.1 93.6,54.74 93.57,54.79 94.56,54.79 94.64,54.81 v94.64,54.79 | R33.1 R27.1 28.5,10.08 | 28.5,10.08 R31.1 R30.1 | 28.5,10.08 v28.5,11.35 | 8.9,20.64 v8.91,20.65 7.24,20.65 5.36,22.52 U7.P5 | USR_SW1.P$4 v1.52,12.29 USR_SW1.P$3 | v14.12,28.3 14.12,29.99 RESET.P$2 21.64,30.02 | RESET.P$1 21.48,30.25 21.42,30.25 21.64,30.02 | 21.72,30.02 21.64,30.02 | C3.2 33.3,27.52 33.3,27.05 35.13,27.05 35.59,27.51 v35.59,27.58 35.59,28.42 35.65,28.35 C46.2 | C16.2 40.92,39.24 40.94,39.05 | R25.2 v34.14,35.74 | 103.52,33.91 U20.P$3 104.83,33.92 v105.08,33.68 | 119.23,27.93 C9.2 119.33,27.74 v119.33,27.05 | v118.95,33.68 119.86,33.68 120.17,33.98 R29.1 | U20.P$55 109.96,36.38 v109.96,38.63 109.96,39.47 C12.2 | 110.87,45.34 v110.8,45.41 109.65,45.41 109.41,45.66 R14.2 105.21,45.66 R13.2 R12.2 | U22.P5 118.44,43.79 v117.42,44.81 | U20.P$39 113.75,30.43 v113.16,31.01 | 40.94,39.05 41.11,39.05 v42.06,38.1 42.44,38.1 U1.P$48 | C44.2 38.26,25.15 v39.32,25.15 | C42.2 57.75,38.26 57.15,38.86 55.24,38.86 v55.02,38.63 55.02,38.41 U1.P$17 | C41.2 40.93,39.05 40.94,39.05 | U5.3 92.96,39.85 94,39.85 | U5.V U5.7 | C40.2 40.54,24.92 40.78,24.67 41.67,24.67 v41.68,24.69 42.06,25.07 42.06,25.46 U1.P$80 | C45.2 39.09,21.03 39.18,20.94 39.91,20.94 v39.93,20.95 | USR_SW2.P$4 v11.25,8.38
  Top 0.152: C8.2 123.05,31.56 123.05,32.32 v122.76,32.61 | U20.P$35 v113.39,28.43 v113.39,28.42 113.39,27.93 U20.P$34 116.41,27.93 C11.2 | C2.2 118.11,27.28 v117.35,26.52 | U20.P$32 112.95,24.36 v113.39,23.93 | U20.P$12 102.5,29.43 v102.18,29.11 101.31,29.11 C13.2 | C5.2 111.11,21.95 v112.01,21.95 | WAKE.P$4 v4.95,34.52 7.85,34.52 7.92,34.44 WAKE.P$3 | U6.P9 117.12,17.75 v116.13,18.75 | U6.P5 116.38,20.07 v116.2,20.04 | U1.P$58 41.21,33.68 v41.91,33.68 | U1.P$55 41.38,35.2 42.06,34.52 v42.67,34.52 | U1.P$10 55.02,34.45 v55.02,34.06 | R34.1 121.08,34.14 121.08,33.38 121.01,33.3 v121.01,32.54 | C33.2 121.16,35.14 v121.16,36.04 | C32.2 7.4,19.74 v8.61,19.74 | R52.1 v8.46,18.59 | USR_SW2.P$3 10.06,15.47 9.98,15.54 v9.98,17.45 | C31.2 17.52,54 | C19.2 91.31,39.78 91.67,39.78 91.59,39.74 C19.2
  Top 0.254: C19.2 91.56,39.81 91.44,39.7 91.59,39.85 92.95,39.85 U5.3 | C20.2 93.46,43.32 v93.88,42.9 | 94,39.85 U5.V | 78.64,43.2 U4.V_4 U4.V | U4.V_2 U4.V_6 U4.V_5 U4.V_3 | v39.4,23.62 39.57,23.6 C4.2 | C15.2 60.33,25.63 v60.5,25.6 | C14.2 59.72,24.41 59.74,24.38 59.78,24.42 59.78,24.34 59.82,24.31 v59.82,24.38 | C29.2 v7.09,6.1 | C30.2 2.67,6.17 3.12,6.17 3.5,6.55 v3.5,7.01 | C6.2 v107.21,40.92 | C7.2 107.52,38.7 v107.52,38.33 | U20.P$27 110.45,24.57 v110.87,24.16 111.98,24.16 111.98,23.2 111.94,23.16 C10.2 | U3.4 118.39,36.55 v118.95,37.11
  Top 0.381: C23.2 64.58,54.56 v65.91,54.56 | C24.2 v65.91,52.12 | C26.2 123.14,47.78 122.91,47.55 v122.3,47.55 | C25.2 v119.41,49.84 | C22.2 33.81,52.48 v33.83,52.5 | C18.2 31.84,36.81 v32.08,36.42 | C17.2 36.93,46.43 v36.88,46.1
  Top 0.406: X11.3 119.82,4.64 119.82,5.45 119.79,5.49 C28.2 C27.2
  Top 0.508: 17.52,54 R47.1 33.58,54 v34.14,54.56
  Bottom 0.152: v28.5,11.35 28.5,11.43 | v8.91,20.65 8.84,20.57 | v59.82,24.38 59.74,24.38 | U21.5 113.06,42.06 v111.33,42.06 | U21.9 U21.3 112.47,45.19 111.71,45.19 111.48,45.41 v110.8,45.41 | v113.16,31.01 113.23,30.94 | v105.08,33.68 105,33.76 | v113.39,28.42 113.46,28.42 | v117.35,26.52 117.42,26.59 | v113.39,23.93 113.46,23.93 | v112.01,21.95 111.94,21.95 | v41.91,33.68 41.83,33.68 | v42.67,34.52 | v8.61,19.74 8.53,19.74 | v8.46,18.59 8.38,18.59 | v9.98,17.45 9.98,17.53 | v34.14,54.56 34.06,54.56
  Bottom 0.254: v93.88,42.9 93.95,42.82 | v39.4,23.62 39.47,23.62 | v7.09,6.1 7.01,6.1 | v107.21,40.92 107.14,40.77 | v107.52,38.33 107.52,38.41 | v110.87,24.16 110.72,24.23 | v118.95,37.11 118.87,37.03
  Bottom 0.381: v65.91,54.56 65.84,54.56 | v65.91,52.12 65.84,52.12 | v119.41,49.84 119.48,49.84 | v33.83,52.5 33.76,52.5 | v32.08,36.42 32.16,36.35
  pour Route2: 0,36.2 29.51,36.2 32.26,38.91 32.26,55.88 124.46,55.88 124.46,0 0,0
ICDI_RESET  (via drill 0.3)
  Top 0.152: U20.P$38 115.14,29.95 116.36,29.95 v116.72,30.31 117.05,29.95 117.88,29.95 118.11,29.72 C2.1 | R3.1 116.36,47.02 115.59,47.78 v114.99,47.78
  Bottom 0.152: v116.72,30.31 115.96,30.31 115.15,30.31 114.91,30.56 114.91,37.41 116.43,38.94 116.43,43.97 116.05,44.35 116.05,44.81 115.82,45.03 115.82,46.94 v114.99,47.78 114.3,47.78 113.39,48.69 112.62,48.69 112.17,48.23 112.17,47.32 112.42,47.07 U21.10
ICDI_TCK  (via drill 0.3)
  Top 0.152: U20.P$52 111.45,38.45 112.32,39.32 112.93,39.32 113.08,39.47 113.08,40.54 113.29,40.77 R4.2 113.29,41.89 113.69,42.29 v114.91,42.29
  Bottom 0.152: U21.4 114.5,42.7 v114.91,42.29
ICDI_TDI  (via drill 0.3)
  Top 0.152: U20.P$50 112.45,37.93 v112.93,38.41
  Bottom 0.152: U21.8 111.63,43.97 111.1,43.43 110.72,43.05 110.72,40.23 112.55,38.41 v112.93,38.41
ICDI_TDO  (via drill 0.3)
  Top 0.152: U20.P$49 112.95,37.54 113.29,37.87 v113.84,37.87
  Bottom 0.152: v113.84,37.87 113.84,38.94 113.23,39.47 113.08,39.62 113.08,40.77 U21.6
ICDI_TMS  (via drill 0.3)
  Top 0.152: U20.P$51 111.95,38.42 112.55,39.01 114.22,39.01 v114.61,38.63 | v115.37,44.42 116.2,44.42 116.22,44.41 116.3,44.41 R5.2
  Bottom 0.152: U21.2 113.74,45.19 115.06,45.19 115.37,44.88 v115.37,44.42 115.37,42.82 115.98,42.22 115.98,39.24 115.37,38.63 v114.61,38.63
ICDI_USBD_N
  Top 0.275: U20.P$43 116.38,32.42 116.43,32.48 117.06,32.48 117.87,33.29 117.87,35.65 U3.2 | 117.87,35.68 U3.2 | U22.P2 119.18,41.84 119.18,41.85 117.44,41.85 116.5,40.91 116.5,38.72 116.97,38.25 117.2,38.25 117.88,37.57 U3.2
ICDI_USBD_P
  Top 0.275: U20.P$44 116.41,32.92 116.43,32.9 116.88,32.9 117.44,33.46 117.44,35.49 117.35,35.59 117.37,35.61 U3.1 117.32,35.74 116.81,35.74 116.51,36.04 116.51,38.1 116.07,38.55 116.07,41.08 117.26,42.28 119.18,42.28 119.39,42.49 U22.P3
ICDI_VDDC
  Top 0.254: C6.1 109.04,40.69 109.12,40.69 109.04,40.62 109.04,40.31 108.8,40.07 C7.1 108.81,39.1 108.81,38.41 109.45,37.76 U20.P$56 109.45,35.24 109.19,34.98 108.66,34.98 108.05,34.37 108.05,32.92 109.45,31.52 U20.P$25 109.45,24.11 109.27,23.93 109.27,22.33 109.58,22.02 109.88,22.02 C5.1
JACK_RX_N
  Top 0.22: U14.6 8.47,47.24 9.93,45.78 11.68,45.78 13.21,47.3 15.54,47.3 | 15.54,47.3 20.47,47.3 | 20.47,47.3 22.25,47.3 22.86,47.91 22.86,49.07 23.29,49.51 U10.P$9 | U13.5 15.6,47.35 15.54,47.3 | U13.4 20.52,47.35 20.47,47.3
JACK_RX_P
  Top 0.22: U14.3 8.71,44.18 9.93,45.41 11.84,45.41 13.36,46.93 15.62,46.93 | 15.62,46.93 20.55,46.93 | 20.55,46.93 24.46,46.93 U10.P$11 | U13.6 15.6,46.91 15.62,46.93 | U13.3 20.52,46.91 20.55,46.93
JACK_TX_N
  Top 0.22: U14.2 9.12,43.16 10.72,44.76 15.52,44.76 | 15.52,44.76 20.65,44.76 | 20.65,44.76 21.84,44.76 23.45,43.16 U10.P$14 | U13.2 20.65,45.21 20.65,44.76 | U13.7 15.52,45.21 15.52,44.76
JACK_TX_P
  Top 0.22: U14.1 8.62,42.14 10.87,44.39 15.57,44.39 | 15.57,44.39 20.62,44.39 | 20.62,44.39 21.69,44.39 22.86,43.22 22.86,41.25 23.5,40.62 U10.P$16 | U13.1 20.62,43.94 20.62,44.39 | U13.8 15.57,43.94 15.57,44.39
MCU_3V3  (via drill 0.3)
  Top 0.152: 55.83,24.41 55.32,24.92 v54.86,24.92 54.9,24.95 54.83,24.95 54.86,25.22 54.86,25.68 54.25,26.29 | 31.47,52.47 C22.1 | v38.56,38.71 37.95,38.71 37.49,39.17 R22.1 37.28,39.3 36.8,39.78 36.68,39.8 R23.1 | v35.43,37.26 35.43,37.34 34.9,37.87 R24.1 34.72,37.97 | C16.1 40.69,40.62 40.79,40.62 C41.1 41.83,39.62 v42.52,38.94 | 39.4,41.07 R21.1 39.24,41.07 38.63,41.68 v38.48,41.68 | 42.75,38.79 v42.52,38.94 | 32.92,22.1 R39.2 32.94,22.25 33.6,22.25 34.29,21.57 36.96,21.57 37.03,21.49 v37.57,21.49 | R2.1 55.67,20.27 56.39,20.27 v56.84,20.73 56.39,21.18 R1.1 | v51.97,21.79 U1.P$101 | 41.57,26.02 arc90 v41.53,25.98 | R41.2 61.91,35.97 v63.09,35.97 | v41.53,25.98 42.02,25.98 U1.P$79 | 41.27,25.98 v41.53,25.98 | 55.63,24.46 55.83,24.41 | 55.83,24.41 C43.1 | C42.1 56.6,38.02 v55.7,38.02 55.19,38.02 U1.P$16 | 42.75,38.94 v42.52,38.94 | C40.1 40.62,25.76 40.83,25.97 41.52,25.97 v41.53,25.98 | U1.P$113 54.25,26.29 | 54.33,26.29 54.25,26.29 | 44.5,41.38 v44.5,41.44 44.5,40.92 44.73,40.92 44.88,40.77 44.88,40.75 U1.P$39 | U1.P$28 51.44,41.05 v51.44,41.91 51.97,41.38 51.97,40.46 U1.P$26 | U1.P$8 55.78,34.08 55.78,33.53 | 55.78,33.53 v55.32,33.07 | U1.P$7 55.79,33.53 55.78,33.53 | U1.P$51 41.38,37.47 v41.38,37.49 41.38,36.91 U1.P$52 | U1.P$69 40.69,30.31 v40.69,30.79 | U1.P$90 46.64,24.38 v46.79,24.54 | U1.P$47 42.82,38.28 42.82,38.63 v42.52,38.94
  Top 0.254: U1.P$122 57.75,27.89 v58.14,27.89
  Top 0.381: C22.1 31.55,52.43 31.55,51.51 32.16,50.9 v33.15,50.9 | U10.P$7 33.05,48.31 v34.52,48.31 | U10.P$2 34.16,41.88 v34.44,41.83 | C18.1 32.73,38.3 32.92,38.48 32.92,39.01 32.93,39.15 v32.92,39.17 | R44.1 25.76,36.12 25.77,36.1 25.77,35.52 v25.38,35.13 | C17.1 36.93,49.33 v36.88,49.38
  Bottom 0.152: v63.09,35.97 63.02,35.97 | v55.7,38.02 55.63,37.95 | v44.5,41.44 44.5,41.45 | v40.69,30.79 40.69,30.71 | v46.79,24.54 46.71,24.38 | v56.84,20.73 56.77,20.8
  Bottom 0.381: v33.15,50.9 33.07,50.9 | v34.52,48.31 34.44,48.31 | v34.44,41.83 34.37,41.91 | v32.92,39.17 32.92,39.09 | v25.38,35.13 25.3,35.13 | v36.88,49.38 36.96,49.38
  pour Route15: 38.94,19.05 55.88,19.05 63.5,26.67 63.5,30.48 66.04,30.48 66.04,33.02 63.5,33.02 63.5,36.83 55.88,44.45 40.64,44.45 40.64,46.76 34.9,52.5 34.9,55.17 32.23,55.17 32.23,38.94 29.49,36.2 24.38,36.2 24.38,32.69 28.12,32.69 33.02,32.64 33.02,26.67 37.49,22.25 37.49,20.5
N$1
  Top 0.152: U20.P$40 114.92,30.94 117.96,30.94 119.18,29.72 119.18,28.95 C9.1 119.48,28.81 120.16,28.81 120.32,28.65 120.51,28.43 Y2.P$1
N$2
  Top 0.152: Y2.P$3 122.53,30.4 122.52,30.42 122.52,31.03 122.3,31.24 122,31.32 C8.1 R50.2
N$3
  Top 0.152: D0.C 92.42,54.76 R9.2
N$4
  Top 0.152: R30.2 D4.C
N$5
  Top 0.152: R31.2 D3.C
N$6
  Top 0.152: D1.C R33.2
N$7  (via drill 0.3)
  Top 0.152: U4.3 77.14,42.09 76.43,41.38 v76.43,40.92 | v76.43,38.94 79.64,38.94 R35.2 79.7,38.02 79.93,37.8 83.52,37.8 84.81,39.09 R26.1
  Bottom 0.152: v76.43,40.92 v76.43,38.94
N$8
  Top 0.152: 5.05,21.6 U7.P$4 | U7.P$6 U7.P$2 U7.P$1 U7.P$5 5.49,19.82 C32.1 R52.2
  Bottom 0.152: U7.P$3 2.7,27.82 U7.P$6 | U7.P$4 2.7,19.82 U7.P$5
N$9
  Top 0.152: 91.43,40.77 C19.1 | 92.96,40.46 U5.2
  Top 0.254: 92.96,40.46 92.35,40.46 92.05,40.69 91.73,40.69 C19.1
  Top 0.305: R48.1 91.35,40.78 91.36,40.77 C19.1
N$10  (via drill 0.3)
  Top 0.152: v83.36,43.89 82.98,43.51 82.45,43.51 82.14,43.2 81.53,43.2 81.38,43.36 80.59,43.36 U4.8 | TP8.TP 81.74,39.14 81.69,39.09 81,39.09 R36.1
  Bottom 0.152: TP8.TP 83.36,40.18 83.36,41.15 83.67,41.45 83.67,42.14 83.36,42.44 v83.36,43.89
N$11
  Top 0.152: C3.1 34.21,28.49 34.21,28.5 R38.2 34.39,28.83 34.44,28.88 34.98,28.88 34.98,29.34 37.41,29.34 37.64,29.11 38.92,29.11 U1.P$68
N$12
  Top 0.152: R40.2 118.62,21.29 U6.P3
N$13
  Top 0.305: 91.67,44.07 C20.1 92.05,43.73 92.05,43.59 92.65,42.99 R48.2 92.66,42.76 92.66,41.91 92.96,41.91 U5.1
  Top 0.381: 91.75,44.03 C20.1 91.68,44.04 90.83,44.04 88.7,41.91 JP3.2
N$14
  Top 0.152: D2.C R27.2
N$15  (via drill 0.3)
  Top 0.152: R29.2 120.17,36.84 R28.1 120.17,35.74 120.05,35.62 119.14,35.62 118.95,35.43 v118.95,34.9 | U20.P$46 116.14,33.92 v116.59,34.37
  Bottom 0.152: v116.59,34.37 118.42,34.37 v118.95,34.9
N$16
  Top 0.152: R49.2 41.15,21.87 41.29,22.01 41.75,22.01 42.22,22.48 44.12,22.48 44.42,22.78 44.48,22.78 U1.P$89
N$17
  Top 0.152: R50.1 119.21,31.43 U20.P$41
N$20
  Top 0.152: U22.P9 121.31,45.99 U22.P10 U22.P7 U22.P6 U22.P11 | U22.P11 121.31,38.99 U22.P8 | U22.P11 122.96,38.95 123.08,38.87 C33.1 R34.2
N$29
  Top 0.152: R49.1 39.09,21.95 38.94,22.1 38.98,22.1 C45.1 38.7,22.1 35.43,22.1 35.26,22.28 35.26,22.66 Y1.P$1
N$30
  Top 0.152: C47.1 28.19,26.52 28.32,26.54 28.17,26.54 28.42,26.52 | 28.42,26.52 28.96,26.52 30.1,27.66 30.1,28.96 31.55,30.4 34.59,30.4 35.36,29.64 37.64,29.64 37.87,29.41 38.68,29.41 38.68,29.43 U1.P$67 | 28.42,26.52 28.34,26.52 27.96,26.67 27.02,26.67 Y3.P$2
N$31
  Top 0.152: 36.27,24.43 Y1.P$3 36.85,24.42 37.11,24.16 38.1,24.16 38.22,24.19 C44.1 | C44.1 38.48,24.17 | C44.1 38.25,24.16 38.18,24.08 38.18,23.47 38.75,22.9 39.44,22.9 39.55,22.78 43.89,22.78 44.42,23.32 44.45,23.32 U1.P$88
N$32
  Top 0.254: U10.P$15 25.7,41.88 26.29,41.3 26.29,40.01 26.14,39.85 23.24,39.85 22.4,40.69 R32.2
N$33
  Top 0.152: 29.26,29.72 30.25,29.72 31.24,30.71 34.82,30.71 35.51,30.02 37.8,30.02 38.1,29.72 38.4,29.72 U1.P$66 | 29.26,29.72 26.29,29.72 26.16,29.59 Y3.P$1 | 29.26,29.72 29.26,29.38 C48.1
N$34
  Top 0.254: U10.P$10 25.91,48.23 26.98,47.17 26.98,39.7 26.67,39.4 22.25,39.4 22.1,39.55 21.64,39.55 R43.2
N$36
  Top 0.254: R45.1 16.3,40.54 | 16.3,40.54 R46.1 | R43.1 20.66,40.53 | 20.66,40.53 20.65,40.54 | 20.66,40.53 20.69,40.5 | 20.69,40.5 R32.1 | 20.69,40.5 20.65,40.77 19.74,40.77 19.51,40.54 19.13,40.54 | 19.13,40.54 16.3,40.54 | C1.1 19.08,40.49 19.13,40.54
N$44
  Top 0.152: U14.4 7.12,45.2 U14.5
  Top 0.254: U14.4 7.07,45.2 6.1,46.18 5.94,46.18 4.65,44.88 4.65,41.99 5.94,40.69 11.73,40.69 12.45,41.4 R45.2
N$45
  Top 0.152: U14.7 7.12,49.28 U14.8
  Top 0.254: U14.8 7.14,49.28 6.1,48.23 6.02,48.23 3.89,46.1 3.89,42.06 5.94,40.01 15.38,40.01 R46.2
PA0  (via drill 0.3)
  Top 0.152: v64.92,26.09 64.95,26.06 67.74,26.06 69.65,24.16 71.93,24.16 72.06,24.18 JP4.2 | v63.27,43.38 62.94,43.05 56.39,43.05 55.85,43.59 50.06,43.59 49.53,43.05 49,43.05 47.49,41.55 U1.P$33 | v63.5,1.75 62.94,2.29 48.08,2.29 47.55,2.82 43.89,2.82 43.59,3.12 42.75,3.12 42.44,2.82 v32.84,2.82 32.99,2.67
  Bottom 0.152: v63.27,43.38 63.25,43.51 63.25,42.06 64.39,40.92 64.39,34.75 63.63,33.98 63.63,33.68 62.79,32.84 62.79,31.85 62.48,31.55 62.48,27.58 64.01,26.06 64.92,26.06 v64.92,26.09 64.92,21.95 63.86,20.8 63.86,6.71 63.55,6.4 63.55,1.83 63.48,1.75 v63.5,1.75 | v32.84,2.82 32.84,2.36 X11.74
PA1  (via drill 0.3)
  Top 0.152: 45.49,44.27 v45.95,44.27 44.35,44.27 44.12,44.04 42.9,44.04 42.29,44.65 38.94,44.65 37.95,43.66 v37.19,43.66 | v69.27,42.22 58.75,42.22 58.22,42.75 55.85,42.75 55.32,43.28 50.22,43.28 49.68,42.75 49.45,42.75 48.54,41.83 48.54,40.92 48.53,40.92 48.23,40.62 47.85,40.62 47.24,41.22 U1.P$34 46.33,42.14 v46.02,42.14
  Bottom 0.152: v46.02,42.14 46.02,42.6 45.95,42.67 v45.95,44.27 | v37.19,43.66 37.19,43.13 36.88,42.82 36.88,40.23 36.12,39.47 36.12,36.96 35.43,36.27 35.43,33.68 34.98,33.22 33.3,33.22 32.16,32.08 32.16,30.56 31.01,29.41 31.01,27.2 29.03,25.22 29.03,14.86 30.02,13.87 30.02,4.8 30.33,4.5 30.33,2.39 X11.76 | JP5.2 71.88,31.75 69.95,33.68 69.95,41.53 v69.27,42.22
PA2  (via drill 0.3)
  Top 0.152: 44,13.56 R20.2 44.04,13.6 44.04,14.02 44.35,14.33 47.47,14.33 47.62,14.48 v49.61,14.48 50.06,14.48 50.29,14.25 52.2,14.25 53.03,13.41 65.68,13.41 66.29,14.02 68.96,14.02 69.65,13.34 v70.56,13.34 | v117.81,6.78 114.38,6.78 114,6.4 113.23,6.4 113.16,6.33 108.89,6.33 108.58,6.02 106.53,6.02 106.22,5.71 97.16,5.71 96.85,6.02 v96.32,6.02 | v96.01,2.59 v71.02,2.59 | U1.P$35 48.31,39.59 v48.31,39.55
  Bottom 0.152: v48.31,39.55 48.31,39.09 48.16,38.94 48.16,34.59 48.92,33.83 48.92,31.47 49.99,30.4 49.99,29.79 49.23,29.03 49.23,25.45 49.91,24.77 49.91,23.55 49.68,23.32 49.68,14.48 v49.61,14.48 | 118.11,1.29 119.18,2.36 119.18,4.42 118.8,4.8 118.8,5.33 117.81,6.33 v117.81,6.78 | v96.32,6.02 96.32,2.9 v96.01,2.59 | v70.56,13.34 70.56,12.88 70.18,12.5 70.18,4.95 71.02,4.12 v71.02,2.59
  Bottom 0.254: 118.11,1.29 X11.6
PA3  (via drill 0.3)
  Top 0.152: v115.14,5.87 115.06,5.79 113.77,5.79 113.69,5.71 109.35,5.71 109.04,5.41 106.98,5.41 106.68,5.11 94.64,5.11 94.49,5.26 93.57,5.26 93.12,4.8 71.86,4.8 71.4,4.34 70.87,4.34 70.18,5.03 69.49,5.03 69.27,4.8 v68.81,4.8 | v68.73,13.26 68.05,13.26 67.82,13.49 66.6,13.49 66.22,13.11 52.88,13.11 52.05,13.95 50.37,13.95 49.61,13.18 v49.23,13.18 48.84,13.56 48.16,13.56 48.12,13.53 48.19,13.38 R19.2 | v46.94,38.63 46.94,39.17 47.32,39.55 47.32,40.01 U1.P$36
  Bottom 0.152: X11.8 115.57,2.31 114.53,3.35 114.53,4.19 115.14,4.8 v115.14,5.87 | v68.81,4.8 68.73,4.88 v68.73,13.26 | v46.94,38.63 46.94,38.1 47.24,37.8 47.24,33.91 48.01,33.15 48.01,28.19 47.4,27.58 47.4,26.36 48.31,25.45 48.31,22.94 49.07,22.17 49.07,16.38 48.31,15.62 48.31,14.1 v49.23,13.18
PA4  (via drill 0.3)
  Top 0.152: v110.11,47.09 109.65,46.63 107.9,46.63 107.59,46.94 90.3,46.94 88.16,44.81 76.96,44.81 75.59,46.18 70.56,46.18 68.66,44.27 62.71,44.27 62.1,43.66 56.84,43.66 56.31,44.2 49.76,44.2 49.23,43.66 46.94,43.66 46.63,43.36 45.41,43.36 | 45.41,43.36 42.06,43.36 41.76,43.66 41.22,43.66 41.17,43.61 v41.22,43.61 | U1.P$37 46.1,40.69 45.41,41.38 45.41,43.36
  Bottom 0.152: v41.22,43.61 41.22,43.66 40.16,44.73 40.16,51.28 X6.18 | X11.10 113.03,2.16 114.22,3.35 114.22,4.12 113.69,4.65 113.69,6.25 114.07,6.63 114.07,35.81 109.73,40.16 109.73,41.83 109.42,42.14 109.42,46.41 109.5,46.48 v110.11,47.09
PA5  (via drill 0.3)
  Top 0.152: v109.04,47.24 90.14,47.24 88.01,45.11 77.19,45.11 75.82,46.48 70.33,46.48 68.43,44.58 62.41,44.58 61.8,43.97 57.15,43.97 56.62,44.5 49.61,44.5 49.07,43.97 46.63,43.97 46.33,43.66 42.52,43.66 41.99,44.2 40.69,44.2 40.46,43.97 | 40.46,43.97 39.7,43.97 v39.29,43.99 | 40.46,43.97 40.46,43.43 40.92,42.98 44.65,42.98 45.11,42.52 45.11,41.07 45.13,41.07 U1.P$38
  Bottom 0.152: X6.20 36.85,52.05 36.85,51.23 39.32,48.77 39.32,44.5 v39.29,43.99 | X11.12 109.5,2.26 109.5,12.95 110.41,13.87 110.41,22.02 109.35,23.09 109.35,24.23 111.1,25.98 111.1,36.35 109.12,38.33 109.12,46.56 109.04,46.63 v109.04,47.24
PA6  (via drill 0.3)
  Top 0.152: X8.16 104.17,50.83 102.41,50.83 101.65,50.06 98.68,50.06 98.37,50.37 v93.88,50.37 93.57,50.06 90.6,50.06 86.87,46.33 78.11,46.33 76.73,47.7 68.73,47.7 67.13,46.1 58.9,46.1 58.37,45.57 55.78,45.57 55.55,45.8 v44.5,45.8 | v44.12,42.37 43.81,42.06 43.81,40.92 44.12,40.62 44.45,40.62 U1.P$40
  Bottom 0.152: v93.88,50.37 92.73,49.23 92.73,25.91 90.98,24.16 90.98,19.58 94.64,15.93 94.64,14.4 93.04,12.8 93.04,5.71 92.73,5.41 92.73,3.83 X11.25 | v44.12,42.37 44.5,42.75 v44.5,45.8
PA7  (via drill 0.3)
  Top 0.152: v90.14,8.15 89.76,8.53 76.89,8.53 76.58,8.23 72.54,8.23 72.24,8.53 v67.59,8.53 66.98,8.53 66.9,8.46 62.56,8.46 62.03,7.85 54.18,7.85 53.14,8.89 X7.8 | v43.2,41 43.97,40.23 44.27,40.23 U1.P$41 | v43.43,45.49 43.74,45.19 44.96,45.19 45.26,45.49 48.84,45.49 49.15,45.19 58.75,45.19 58.98,45.49 v65.46,45.49
  Bottom 0.152: X11.27 90.14,3.83 v90.14,8.15 | v43.2,41 43.2,42.52 43.51,42.82 43.51,44.5 43.43,44.58 v43.43,45.49 | v65.46,45.49 65.46,36.5 68.66,33.3 68.66,28.19 67.97,27.51 67.97,15.24 67.74,15.01 67.74,12.88 67.89,12.72 67.89,12.34 67.74,12.19 67.74,9.14 67.59,8.99 v67.59,8.53
PB0  (via drill 0.3)
  Top 0.152: v54.79,6.02 54.48,5.79 48.31,5.79 48.23,5.71 42.67,5.71 42.6,5.79 v41.3,5.79 41.22,5.87 | R18.1 18.94,22.63 26.36,22.63 30.79,18.21 36.04,18.21 37.26,19.43 41.76,19.43 v42.06,19.74 43.43,21.11 46.18,21.11 47.19,22.12 U1.P$95
  Bottom 0.152: X11.58 52.07,2.16 53.42,3.5 53.42,4.19 54.79,5.56 v54.79,6.02 | v41.3,5.79 39.93,7.16 39.93,7.92 40.46,8.46 40.46,11.51 41.53,12.57 41.53,13.49 41.15,13.87 41.15,16.08 42.06,16.99 v42.06,19.74
PB2  (via drill 0.3)
  Top 0.152: X8.17 102.62,54.61 101.58,53.57 92.2,53.57 v91.44,52.81 | v91.44,51.51 90.22,51.51 85.95,47.24 78.79,47.24 76.5,49.53 67.97,49.53 66.14,47.7 55.24,47.7 54.79,47.32 v47.55,47.32 v38.56,47.32 | v48.31,26.75 48.31,25.07 47.17,23.93 46.79,23.93 46.25,23.39 46.22,23.39 U1.P$91 | v38.71,5.49 v36.2,5.49
  Bottom 0.152: v91.44,52.81 v91.44,51.51 | v47.55,47.32 47.55,44.2 48.46,43.28 48.46,41.15 47.55,40.23 47.55,39.4 47.85,39.09 47.85,34.37 48.62,33.6 48.62,27.81 48.31,27.51 v48.31,26.75 | X11.67 39.37,4.85 v38.71,5.49 | v36.2,5.49 35.2,6.48 35.2,7.7 35.51,8 35.51,10.82 35.81,11.12 35.81,26.82 36.35,27.36 36.35,27.81 35.36,28.8 35.36,31.17 36.2,32 36.2,36.04 36.73,36.58 36.73,39.09 37.49,39.85 37.49,42.14 38.1,42.75 38.1,44.88 37.87,45.11 37.87,46.63 v38.56,47.32
PB3  (via drill 0.3)
  Top 0.152: X8.19 95.45,54.61 94.79,53.95 91.67,53.95 85.57,47.85 79.32,47.85 77.04,50.14 67.36,50.14 65.53,48.31 54.63,48.31 54.56,48.23 47.09,48.23 46.79,48.54 v46.33,48.54 46.02,48.23 43.97,48.23 43.59,48.62 v38.48,48.62 | v49,24 48.54,24 48.16,23.62 47.01,23.62 U1.P$92
  Bottom 0.152: v46.33,48.54 46.33,44.88 48.08,43.13 48.08,41.38 47.24,40.54 47.24,39.24 47.55,38.94 47.55,34.14 48.31,33.38 48.31,28.04 47.7,27.43 47.7,26.52 48.62,25.6 48.62,25.07 49,24.69 v49,24 | X11.69 36.83,3.86 35.36,5.33 35.05,5.33 34.44,5.94 34.44,7.47 35.13,8.15 35.13,11.2 35.43,11.51 35.43,26.21 34.9,26.75 34.9,31.39 35.81,32.31 35.81,36.2 36.42,36.8 36.42,39.24 37.19,40.01 37.19,42.44 37.8,43.05 37.8,44.65 37.57,44.88 37.57,47.7 v38.48,48.62
PB4  (via drill 0.3)
  Top 0.152: v94.03,12.65 v78.56,12.65 | v94.03,4.65 94.56,4.65 94.72,4.8 106.91,4.8 107.21,5.11 109.19,5.11 109.5,5.41 113.92,5.41 114,5.49 114.68,5.49 114.91,5.26 117.65,5.26 v117.81,5.41 | v78.56,26.75 76.5,26.75 75.29,27.96 71.25,27.96 70.56,27.28 57.84,27.28 57.07,28.04 57.03,28.04 U1.P$121 55.85,29.21 55.85,29.87 56.24,30.25 v56.24,30.94
  Bottom 0.152: v78.56,12.65 78.56,17.6 78.87,17.91 78.87,20.04 78.56,20.34 v78.56,26.75 | v94.03,12.65 v94.03,4.65 | v117.81,5.41 117.81,4.95 118.11,4.65 X11.5 | X6.6 54.61,50.88 53.87,50.14 53.87,44.27 54.41,43.74 54.41,33.07 56.24,31.24 v56.24,30.94
PB5  (via drill 0.3)
  Top 0.152: v116.05,5.87 116.05,6.48 114.83,6.48 114.45,6.1 113.46,6.1 113.39,6.02 109.12,6.02 108.81,5.71 106.76,5.71 106.45,5.41 94.87,5.41 94.72,5.56 93.34,5.56 93.19,5.41 86.87,5.41 86.56,5.11 71.25,5.11 v71.09,5.03 | v69.57,26.67 68.5,26.67 68.2,26.98 57.68,26.98 56.92,27.74 56.77,27.74 U1.P$120 55.47,29.03 55.47,30.1 v54.71,30.86
  Bottom 0.152: X11.7 115.57,5.38 v116.05,5.87 | v71.09,5.03 71.09,8.38 71.48,8.76 71.48,20.88 70.56,21.79 70.56,23.62 71.09,24.16 71.09,25.15 v69.57,26.67 | X6.8 52.07,51.03 52.88,50.22 52.88,43.74 53.49,43.13 53.49,32.16 v54.71,30.86
PC4  (via drill 0.3)  (1 unrouted)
